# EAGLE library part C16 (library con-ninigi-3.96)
NINIGI
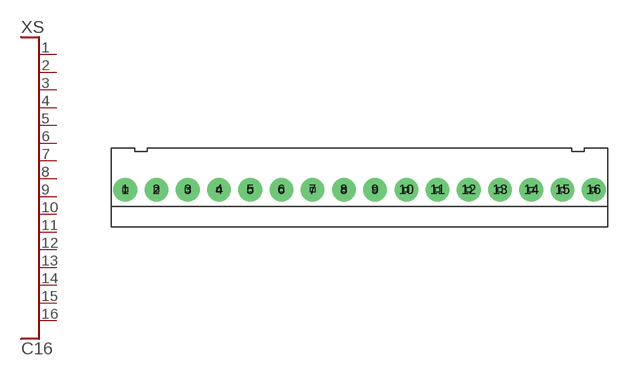
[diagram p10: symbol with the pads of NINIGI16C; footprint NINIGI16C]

Designator prefix XS

## C16  [NINIGI16C]
1  P$1
2  P$2
3  P$3
4  P$4
5  P$5
6  P$6
7  P$7
8  P$8
9  P$9
10  P$10
11  P$11
12  P$12
13  P$13
14  P$14
15  P$15
16  P$16

## Footprint NINIGI16C (pad centres in mm)
drill 1.6 pad 3: 1 -29.7,0; 2 -25.74,0; 3 -21.78,0; 4 -17.82,0; 5 -13.86,0; 6 -9.9,0; 7 -5.94,0; 8 -1.98,0; 9 1.98,0; 10 5.94,0; 11 9.9,0; 12 13.86,0; 13 17.82,0; 14 21.78,0; 15 25.74,0; 16 29.7,0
